|   stm32f0_444_lqfp48 IBIS Model
[IBIS ver]   4.2
[File name]  stm32f0_444_lqfp48.ibs
[File Rev]   1.0
[Date]   15-5-2013
[Source] Data Created at STMicroelectronics
[Notes]   File originated from ELDO simulations.
[Disclaimer]  This information is for modeling purpose only and is
   not guaranted. The information is subject to change without
   notice.
[Copyright] Copyright 2015 STMicroelectronics Inc.
[Component] stm32f0_444_lqfp48
[Manufacturer] STMicroelectronics
[Package]
| variable   typ   min   max
R_pkg   0.0   NA   NA
L_pkg   0.0H   NA   NA
C_pkg   0.0F   NA   NA
[Pin] signal_name  model_name   R_pin   L_pin   C_pin
1   VBAT   POWER   69.0E-3   4.2E-9   120.0E-15
2   PC13   io8p_sudq_tc   61.9E-3   3.5E-9   84.0E-15
3   PC14   io8p_sudq_tc   56.4E-3   2.9E-9   56.0E-15
4   PC15   io8p_sudq_tc   52.4E-3   2.5E-9   36.0E-15
5   PF0   io8p_sudq_ft   50.1E-3   2.3E-9   24.0E-15
6   PF1   io8p_sudq_ft   49.3E-3   2.2E-9   20.0E-15
7   NRST   ioreset_tc_v33   49.3E-3   2.2E-9   20.0E-15
8   VSSA   GND   50.1E-3   2.3E-9   24.0E-15
9   VDDA   POWER   52.4E-3   2.5E-9   36.0E-15
10   PA0   io8p_sudq_ft   56.4E-3   2.9E-9   56.0E-15
11   PA1   io8p_sudq_ft   61.9E-3   3.5E-9   84.0E-15
12   PA2   io8p_sudq_ft   69.0E-3   4.2E-9   120.0E-15
13   PA3   io8p_sudq_ft   69.0E-3   4.2E-9   120.0E-15
14   PA4   io8p_sudq_ft   61.9E-3   3.5E-9   84.0E-15
15   PA5   io8p_sudq_ft   56.4E-3   2.9E-9   56.0E-15
16   PA6   io8p_sudq_ft   52.4E-3   2.5E-9   36.0E-15
17   PA7   io8p_sudq_ft   50.1E-3   2.3E-9   24.0E-15
18   PB0   io8p_sudq_ft   49.3E-3   2.2E-9   20.0E-15
19   PB1   io8p_sudq_ft   49.3E-3   2.2E-9   20.0E-15
20   PB2   io8p_sudq_ft   50.1E-3   2.3E-9   24.0E-15
21   PB10   io8p_sudq_i2cin_lv_ft   52.4E-3   2.5E-9   36.0E-15
22   PB11   io8p_sudq_i2cin_lv_ft   56.4E-3   2.9E-9   56.0E-15
23   VSS   GND   61.9E-3   3.5E-9   84.0E-15
24   VDD   POWER   69.0E-3   4.2E-9   120.0E-15
25   PB12   io8p_sudq_ft   69.0E-3   4.2E-9   120.0E-15
26   PB13   io8p_sudq_ft   61.9E-3   3.5E-9   84.0E-15
27   PB14   io8p_sudq_ft   56.4E-3   2.9E-9   56.0E-15
28   PB15   io8p_sudq_ft   52.4E-3   2.5E-9   36.0E-15
29   PA8   io8p_sudq_ft   50.1E-3   2.3E-9   24.0E-15
30   PA9   io8p_sudq_ft   49.3E-3   2.2E-9   20.0E-15
31   PA10   io8p_sudq_ft   49.3E-3   2.2E-9   20.0E-15
32   PA11   io8p_sudq_ft   50.1E-3   2.3E-9   24.0E-15
33   PA12   io8p_sudq_ft   52.4E-3   2.5E-9   36.0E-15
34   PA13   io8p_sudq_ft   56.4E-3   2.9E-9   56.0E-15
35   PF6   io8p_sudq_i2cin_lv_ft   61.9E-3   3.5E-9   84.0E-15
36   PF7   io8p_sudq_i2cin_lv_ft   69.0E-3   4.2E-9   120.0E-15
37   PA14   io8p_sudq_ft   69.0E-3   4.2E-9   120.0E-15
38   PA15   io8p_sudq_ft   61.9E-3   3.5E-9   84.0E-15
39   PB3   io8p_sudq_ft   56.4E-3   2.9E-9   56.0E-15
40   PB4   io8p_sudq_ft   52.4E-3   2.5E-9   36.0E-15
41   PB5   io8p_sudq_ft   50.1E-3   2.3E-9   24.0E-15
42   PB6   io8p_sudq_i2cin_lv_ft   49.3E-3   2.2E-9   20.0E-15
43   PB7   io8p_sudq_i2cin_lv_ft   49.3E-3   2.2E-9   20.0E-15
44   BOOT0   vpp_test_hv   50.1E-3   2.3E-9   24.0E-15
45   PB8   io8p_sudq_i2cin_lv_ft   52.4E-3   2.5E-9   36.0E-15
46   PB9   io8p_sudq_i2cin_lv_ft   56.4E-3   2.9E-9   56.0E-15
47   VSS   GND   61.9E-3   3.5E-9   84.0E-15
48   VDD   POWER   69.0E-3   4.2E-9   120.0E-15
[Model Selector] io8p_sudq_ft
io8p01_sudq_ft_pd_lv  "SPEED01 2P0V, PD=40kOhm"
io8p01_sudq_ft_pu_lv  "SPEED01 2P0V, PU=40kOhm"
io8p01_sudq_ft_lv  "SPEED01 2P0V"
io8p10_sudq_ft_pd_lv  "SPEED10 2P0V, PD=40kOhm"
io8p10_sudq_ft_pu_lv  "SPEED10 2P0V, PU=40kOhm"
io8p10_sudq_ft_lv  "SPEED10 2P0V"
io8p11_sudq_ft_pd_lv  "SPEED11 2P0V, PD=40kOhm"
io8p11_sudq_ft_pu_lv  "SPEED11 2P0V, PU=40kOhm"
io8p11_sudq_ft_lv  "SPEED11 2P0V"
io8p01_sudq_ft_pd  "SPEED01, PD=40kOhm"
io8p01_sudq_ft_pu  "SPEED01, PU=40kOhm"
io8p01_sudq_ft  "SPEED01"
io8p10_sudq_ft_pd  "SPEED10, PD=40kOhm"
io8p10_sudq_ft_pu  "SPEED10, PU=40kOhm"
io8p10_sudq_ft  "SPEED10"
io8p11_sudq_ft_pd  "SPEED11, PD=40kOhm"
io8p11_sudq_ft_pu  "SPEED11, PU=40kOhm"
io8p11_sudq_ft  "SPEED11"
[Model Selector] io8p_sudq_i2cin_lv_ft
io8p01_sudq_i2cin_lv_ft_pd_lv  "SPEED01 2P0V, PD=40kOhm"
io8p01_sudq_i2cin_lv_ft_pu_lv  "SPEED01 2P0V, PU=40kOhm"
io8p01_sudq_i2cin_lv_ft_lv  "SPEED01 2P0V"
io8p10_sudq_i2cin_lv_ft_pd_lv  "SPEED10 2P0V, PD=40kOhm"
io8p10_sudq_i2cin_lv_ft_pu_lv  "SPEED10 2P0V, PU=40kOhm"
io8p10_sudq_i2cin_lv_ft_lv  "SPEED10 2P0V"
io8p11_sudq_i2cin_lv_ft_pd_lv  "SPEED11 2P0V, PD=40kOhm"
io8p11_sudq_i2cin_lv_ft_pu_lv  "SPEED11 2P0V, PU=40kOhm"
io8p11_sudq_i2cin_lv_ft_lv  "SPEED11 2P0V"
io8p01_sudq_i2cin_lv_ft_pd  "SPEED01, PD=40kOhm"
io8p01_sudq_i2cin_lv_ft_pu  "SPEED01, PU=40kOhm"
io8p01_sudq_i2cin_lv_ft  "SPEED01"
io8p10_sudq_i2cin_lv_ft_pd  "SPEED10, PD=40kOhm"
io8p10_sudq_i2cin_lv_ft_pu  "SPEED10, PU=40kOhm"
io8p10_sudq_i2cin_lv_ft  "SPEED10"
io8p11_sudq_i2cin_lv_ft_pd  "SPEED11, PD=40kOhm"
io8p11_sudq_i2cin_lv_ft_pu  "SPEED11, PU=40kOhm"
io8p11_sudq_i2cin_lv_ft  "SPEED11"
[Model Selector] io8p_sudq_tc
io8p01_sudq_tc_pd_lv  "SPEED01 2P0V, PD=40kOhm"
io8p01_sudq_tc_pu_lv  "SPEED01 2P0V, PU=40kOhm"
io8p01_sudq_tc_lv  "SPEED01 2P0V"
io8p10_sudq_tc_pd_lv  "SPEED10 2P0V, PD=40kOhm"
io8p10_sudq_tc_pu_lv  "SPEED10 2P0V, PU=40kOhm"
io8p10_sudq_tc_lv  "SPEED10 2P0V"
io8p11_sudq_tc_pd_lv  "SPEED11 2P0V, PD=40kOhm"
io8p11_sudq_tc_pu_lv  "SPEED11 2P0V, PU=40kOhm"
io8p11_sudq_tc_lv  "SPEED11 2P0V"
io8p01_sudq_tc_pd  "SPEED01, PD=40kOhm"
io8p01_sudq_tc_pu  "SPEED01, PU=40kOhm"
io8p01_sudq_tc  "SPEED01"
io8p10_sudq_tc_pd  "SPEED10, PD=40kOhm"
io8p10_sudq_tc_pu  "SPEED10, PU=40kOhm"
io8p10_sudq_tc  "SPEED10"
io8p11_sudq_tc_pd  "SPEED11, PD=40kOhm"
io8p11_sudq_tc_pu  "SPEED11, PU=40kOhm"
io8p11_sudq_tc  "SPEED11"
[Model Selector] ioreset_tc_v33
ioreset_tc_v33_pu_lv  "IORESET 2V + PU=40kOhm"
ioreset_tc_v33_nopu_lv  "IORESET 2V"
ioreset_tc_v33_pu  "IORESET + PU=40kOhm"
ioreset_tc_v33_nopu  "IORESET"
[Model Selector] vpp_test_hv
vpp_test_hv_3p3  "Input Buffer"
vpp_test_hv_2p4  "Input Buffer 2P0V"
| Models and submodels in the file (60): io8p01_sudq_ft_pd_lv (I/O), io8p01_sudq_ft_pu_lv (I/O), io8p01_sudq_ft_lv (I/O), io8p10_sudq_ft_pd_lv (I/O), io8p10_sudq_ft_pu_lv (I/O), io8p10_sudq_ft_lv (I/O), io8p11_sudq_ft_pd_lv (I/O), io8p11_sudq_ft_pu_lv (I/O), io8p11_sudq_ft_lv (I/O), io8p01_sudq_ft_pd (I/O), io8p01_sudq_ft_pu (I/O), io8p01_sudq_ft (I/O), io8p10_sudq_ft_pd (I/O), io8p10_sudq_ft_pu (I/O), io8p10_sudq_ft (I/O), io8p11_sudq_ft_pd (I/O), io8p11_sudq_ft_pu (I/O), io8p11_sudq_ft (I/O), io8p01_sudq_i2cin_lv_ft_pd_lv (I/O), io8p01_sudq_i2cin_lv_ft_pu_lv (I/O), io8p01_sudq_i2cin_lv_ft_lv (I/O), io8p10_sudq_i2cin_lv_ft_pd_lv (I/O), io8p10_sudq_i2cin_lv_ft_pu_lv (I/O), io8p10_sudq_i2cin_lv_ft_lv (I/O), io8p11_sudq_i2cin_lv_ft_pd_lv (I/O), io8p11_sudq_i2cin_lv_ft_pu_lv (I/O), io8p11_sudq_i2cin_lv_ft_lv (I/O), io8p01_sudq_i2cin_lv_ft_pd (I/O), io8p01_sudq_i2cin_lv_ft_pu (I/O), io8p01_sudq_i2cin_lv_ft (I/O), io8p10_sudq_i2cin_lv_ft_pd (I/O), io8p10_sudq_i2cin_lv_ft_pu (I/O), io8p10_sudq_i2cin_lv_ft (I/O), io8p11_sudq_i2cin_lv_ft_pd (I/O), io8p11_sudq_i2cin_lv_ft_pu (I/O), io8p11_sudq_i2cin_lv_ft (I/O), io8p01_sudq_tc_pd_lv (I/O), io8p01_sudq_tc_pu_lv (I/O), io8p01_sudq_tc_lv (I/O), io8p10_sudq_tc_pd_lv (I/O), io8p10_sudq_tc_pu_lv (I/O), io8p10_sudq_tc_lv (I/O), io8p11_sudq_tc_pd_lv (I/O), io8p11_sudq_tc_pu_lv (I/O), io8p11_sudq_tc_lv (I/O), io8p01_sudq_tc_pd (I/O), io8p01_sudq_tc_pu (I/O), io8p01_sudq_tc (I/O), io8p10_sudq_tc_pd (I/O), io8p10_sudq_tc_pu (I/O), io8p10_sudq_tc (I/O), io8p11_sudq_tc_pd (I/O), io8p11_sudq_tc_pu (I/O), io8p11_sudq_tc (I/O), ioreset_tc_v33_pu_lv (I/O_open_drain), ioreset_tc_v33_nopu_lv (I/O_open_drain), ioreset_tc_v33_pu (I/O_open_drain), ioreset_tc_v33_nopu (I/O_open_drain), vpp_test_hv_2p4 (Input), vpp_test_hv_3p3 (Input)
